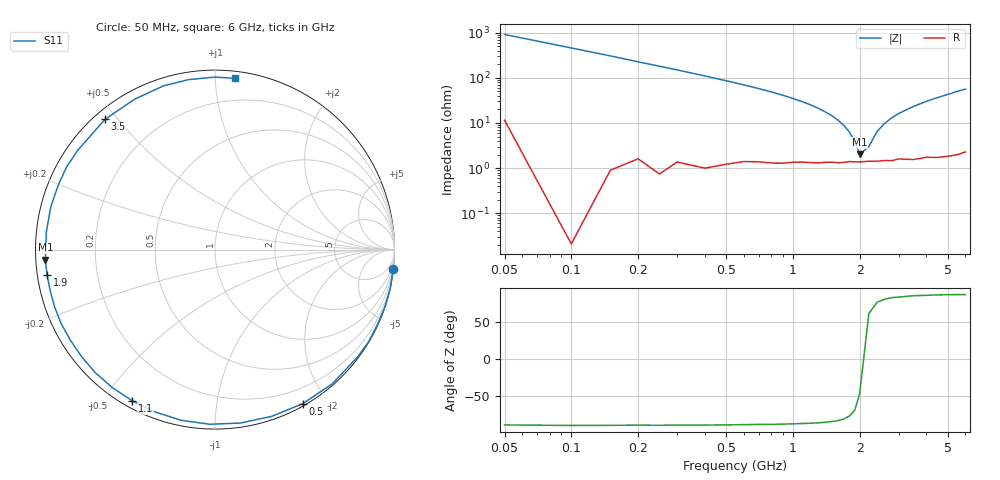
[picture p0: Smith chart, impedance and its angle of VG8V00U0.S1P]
! Infineon Technologies  Discrete & RF Semiconductors
! BB 831
! Si Tuning Diode in SOD323
! VR = 8 V
! S-Parameters:  July  1999
# GHz  S  MA  R  50
!  f  S11
! GHz  MAG  ANG
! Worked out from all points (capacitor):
!   34 points, 50 MHz to 6 GHz, reference 50 ohm
!   read as one part to ground: C = 3.48 pF near 50 MHz
!   lowest |Z| = 2.02 ohm at 2 GHz (marker M1)
!   series resonance near 2.072 GHz, so ESL is about 1.7 nH
!   S11 on the Smith chart (normalised r, x): 50 MHz: 0, -18; 500 MHz: 0.02, -1.72; 1.1 GHz: 0.03, -0.59; 1.9 GHz: 0.03, -0.07; 3.5 GHz: 0.03, +0.46; 6 GHz: 0.05, +1.12
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0.05  0.9986 -6.3
0.15  0.9991 -18.6
0.25  0.9979 -31.0
0.4  0.9932 -48.9
0.5  0.9877 -60.4
0.6  0.9811 -71.3
0.7  0.9766 -81.7
0.8  0.9736 -91.7
0.9  0.9696 -101.2
1  0.9642 -110.2
1.1  0.9604 -118.6
1.2  0.9585 -126.5
1.3  0.9566 -134.1
1.4  0.9531 -141.3
1.6  0.9512 -154.3
1.7  0.9491 -160.4
1.9  0.9465 -171.5
2  0.9464 -176.6
2.2  0.9448 173.9
2.4  0.9453 165.5
2.6  0.9447 157.7
3  0.9437 144.2
3.5  0.9501 130.2
4  0.9501 118.0
4.5  0.956 107.6
5  0.9585 98.8
5.5  0.9611 90.1
6  0.9604 83.3
